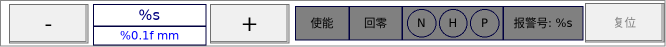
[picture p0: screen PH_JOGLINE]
VISUALIZATION PH_JOGLINE  // 666x47
VAR_IN_OUT
	m_Input_Name : Axis_PTP_CoE;
END_VAR
    RoundedRectangle (402,6 101x34)
    Rectangle (93,4 113x22), "%s", text variable: m_Input_Name.sName, text list: ''
    Button (210,4 79x39), "+"
        tap m_Input_Name.IO.btManualJogF
    Rectangle (93,26 113x19), "%0.1f mm", text variable: m_Input_Name.Ref.NcToPlc.ActPos, colour toggle: (m_Input_Name.Ref.Status.Moving) <> 0
    Button (9,4 79x39), "-"
        tap m_Input_Name.IO.btManualJogB
    RoundedRectangle (295,6 54x34), "使能", colour toggle: (m_Input_Name.Ref.Status.ControlLoopClosed) <> 0
    RoundedRectangle (349,6 53x34), "回零", colour toggle: (m_Input_Name.Ref.Status.Homed) <> 0
    RoundedRectangle (503,6 80x34), "报警号: %s", text variable: m_Input_Name.Ref.Status.ErrorID, colour toggle: (m_Input_Name.Ref.Status.Error) <> 0
    Ellipse (407,9 29x28), "N", colour toggle: (m_Input_Name.IO.snLimitN) <> 0
    Ellipse (470,9 29x28), "P", colour toggle: (m_Input_Name.IO.snLimitP) <> 0
    Ellipse (439,9 28x28), "H", colour toggle: (m_Input_Name.IO.snHome) <> 0
    Button (585,3 79x39), "复位"
        tap m_Input_Name.bReset
END_VISUALIZATION
